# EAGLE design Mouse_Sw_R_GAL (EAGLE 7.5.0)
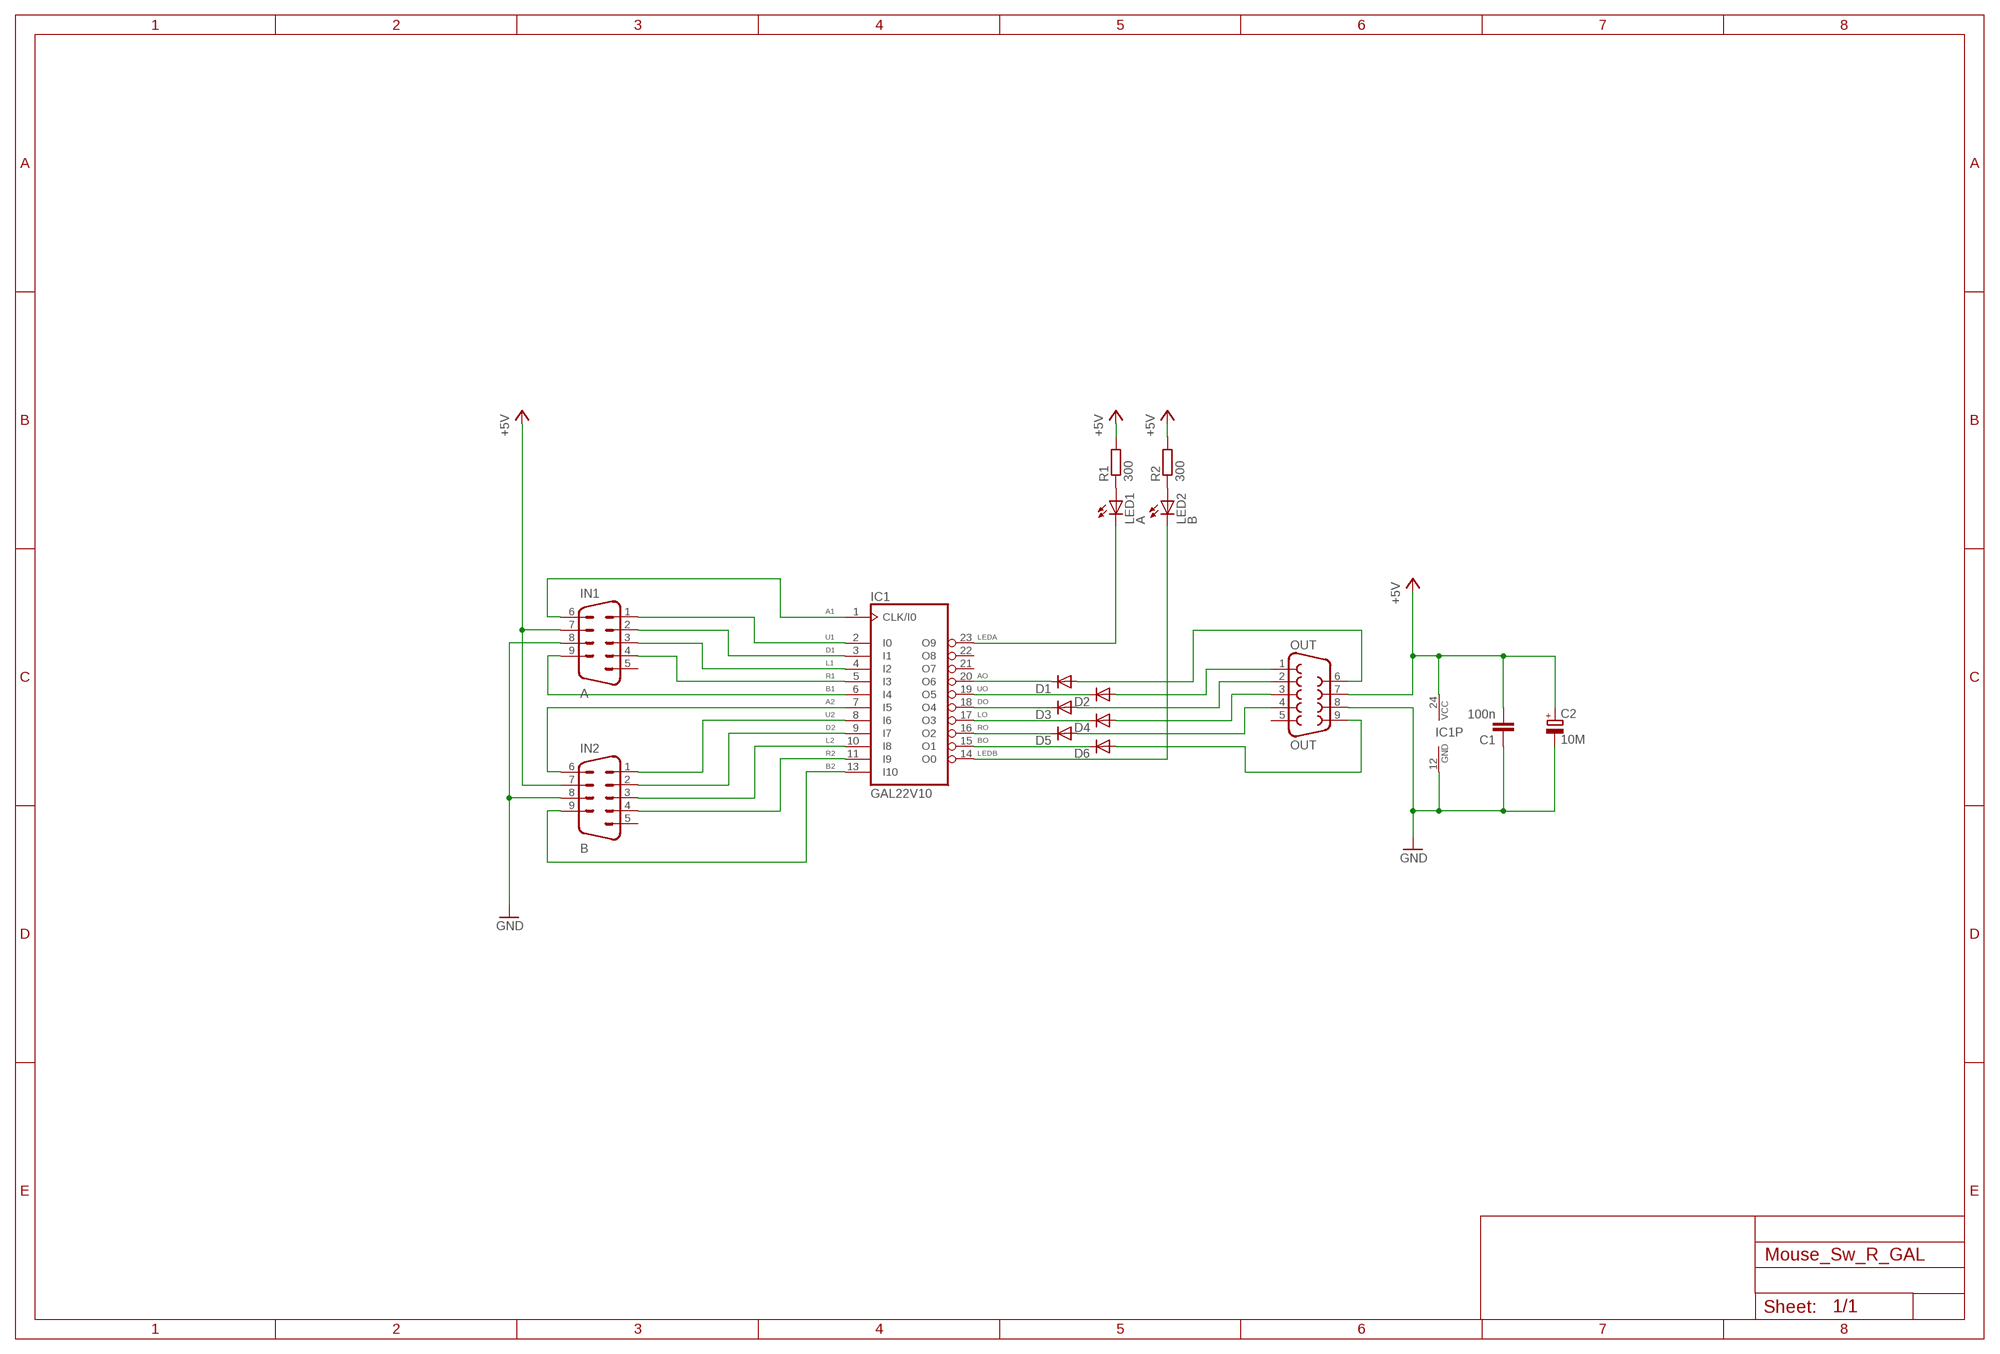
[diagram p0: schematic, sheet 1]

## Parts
C1  100n  C-EU050-024X044  [C050-024X044]
C2  10M  CPOL-EUE2.5-5  [E2,5-5]
D1  DIODE-D-5  [D-5]
D2  DIODE-D-5  [D-5]
D3  DIODE-D-5  [D-5]
D4  DIODE-D-5  [D-5]
D5  DIODE-D-5  [D-5]
D6  DIODE-D-5  [D-5]
IC1  GAL22V10  22V10  [DIL24-3]
IN1  A  M09D  [M09D]
IN2  B  M09D  [M09D]
LED1  A  LED3MM  [LED3MM]
LED2  B  LED3MM  [LED3MM]
OUT  OUT  F09D  [F09D]
R1  300  R-EU_0204/5  [0204/5]
R2  300  R-EU_0204/5  [0204/5]

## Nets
+5V: C1.2 C2.+ IC1.24(VCC) IN1.7 IN2.7 OUT.7 R1.2 R2.2
A: D1.A OUT.6
A1: IC1.1(CLK/I0) IN1.6
A2: IC1.7(I5) IN2.6
AO: D1.C IC1.20(O6)
B: D6.A OUT.9
B1: IC1.6(I4) IN1.9
B2: IC1.13(I10) IN2.9
BO: D6.C IC1.15(O1)
D: D3.A OUT.2
D1: IC1.3(I1) IN1.2
D2: IC1.9(I7) IN2.2
DO: D3.C IC1.18(O4)
GND: C1.1 C2.- IC1.12(GND) IN1.8 IN2.8 OUT.8
L: D4.A OUT.3
L1: IC1.4(I2) IN1.3
L2: IC1.10(I8) IN2.3
LEDA: IC1.23(O9) LED1.K(C)
LEDB: IC1.14(O0) LED2.K(C)
LO: D4.C IC1.17(O3)
N$22: LED1.A R1.1
N$29: LED2.A R2.1
R: D5.A OUT.4
R1: IC1.5(I3) IN1.4
R2: IC1.11(I9) IN2.4
RO: D5.C IC1.16(O2)
U: D2.A OUT.1
U1: IC1.2(I0) IN1.1
U2: IC1.8(I6) IN2.1
UO: D2.C IC1.19(O5)
Unconnected: IC1.21(O7) IC1.22(O8) IN1.5 IN2.5 OUT.5

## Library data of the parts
C1 = rcl:C-EU: CAPACITOR, European symbol
C2 = rcl:CPOL-EU: POLARIZED CAPACITOR, European symbol
D1-D6 = diode:DIODE-: DIODE
IC1 = pal:22V10: PAL; MPN: GAL22V10D-7LPN; OC_FARNELL: 1571925; OC_NEWARK: 97M0480
IN1 IN2 = con-subd:M09: SUB-D; OC_FARNELL: unknown; OC_NEWARK: unknown
LED1 LED2 = led:LED: LED
OUT = con-subd:F09: SUB-D; OC_FARNELL: unknown; OC_NEWARK: unknown
R1 R2 = rcl:R-EU_: RESISTOR, European symbol

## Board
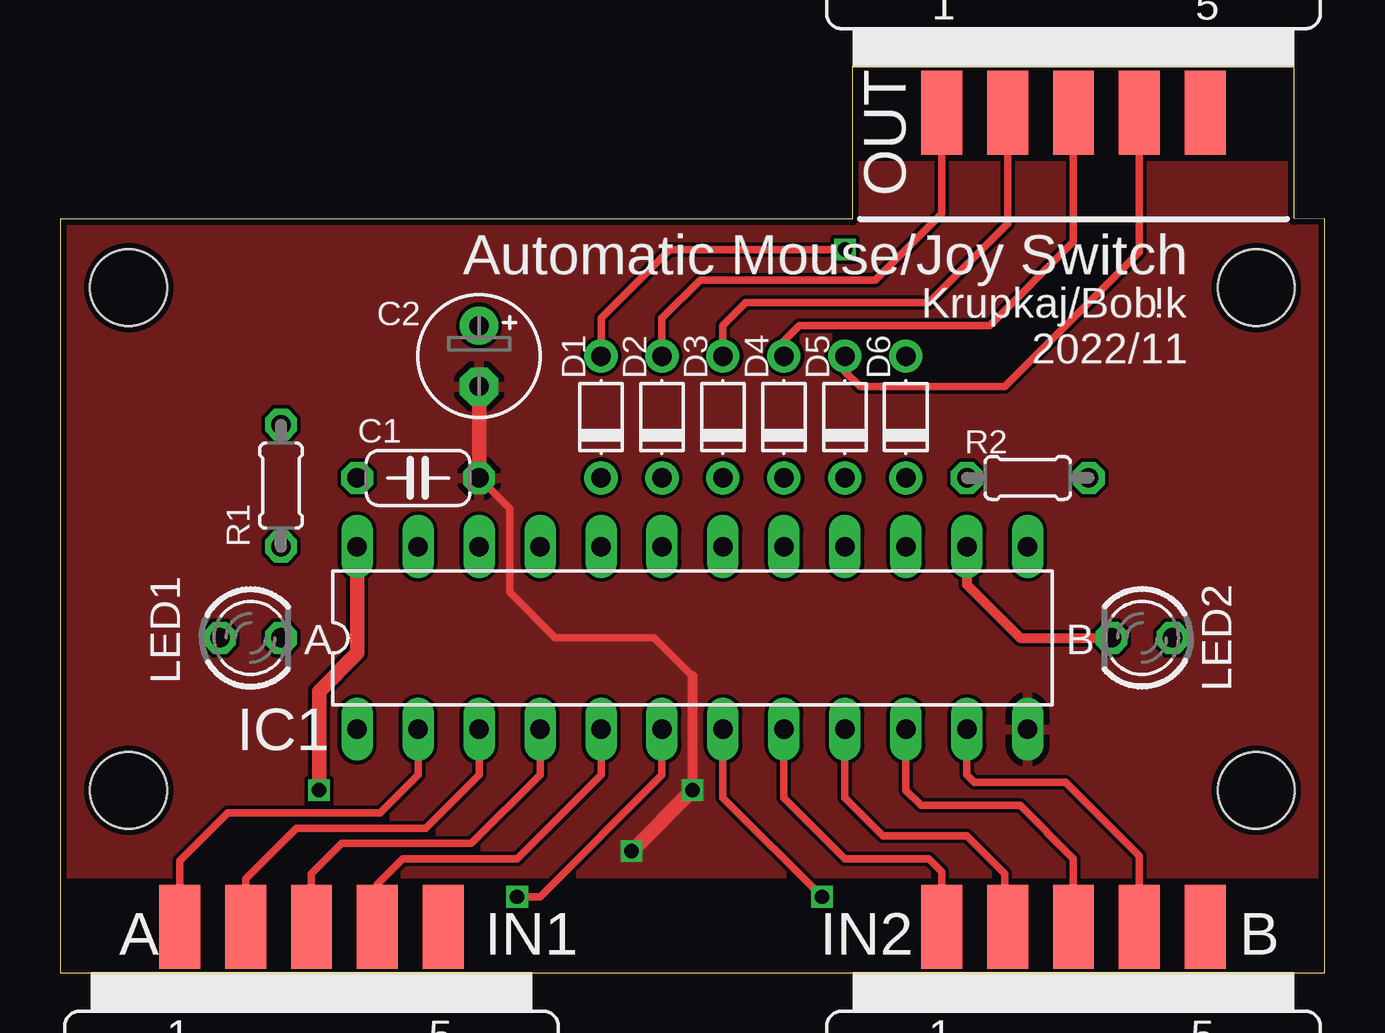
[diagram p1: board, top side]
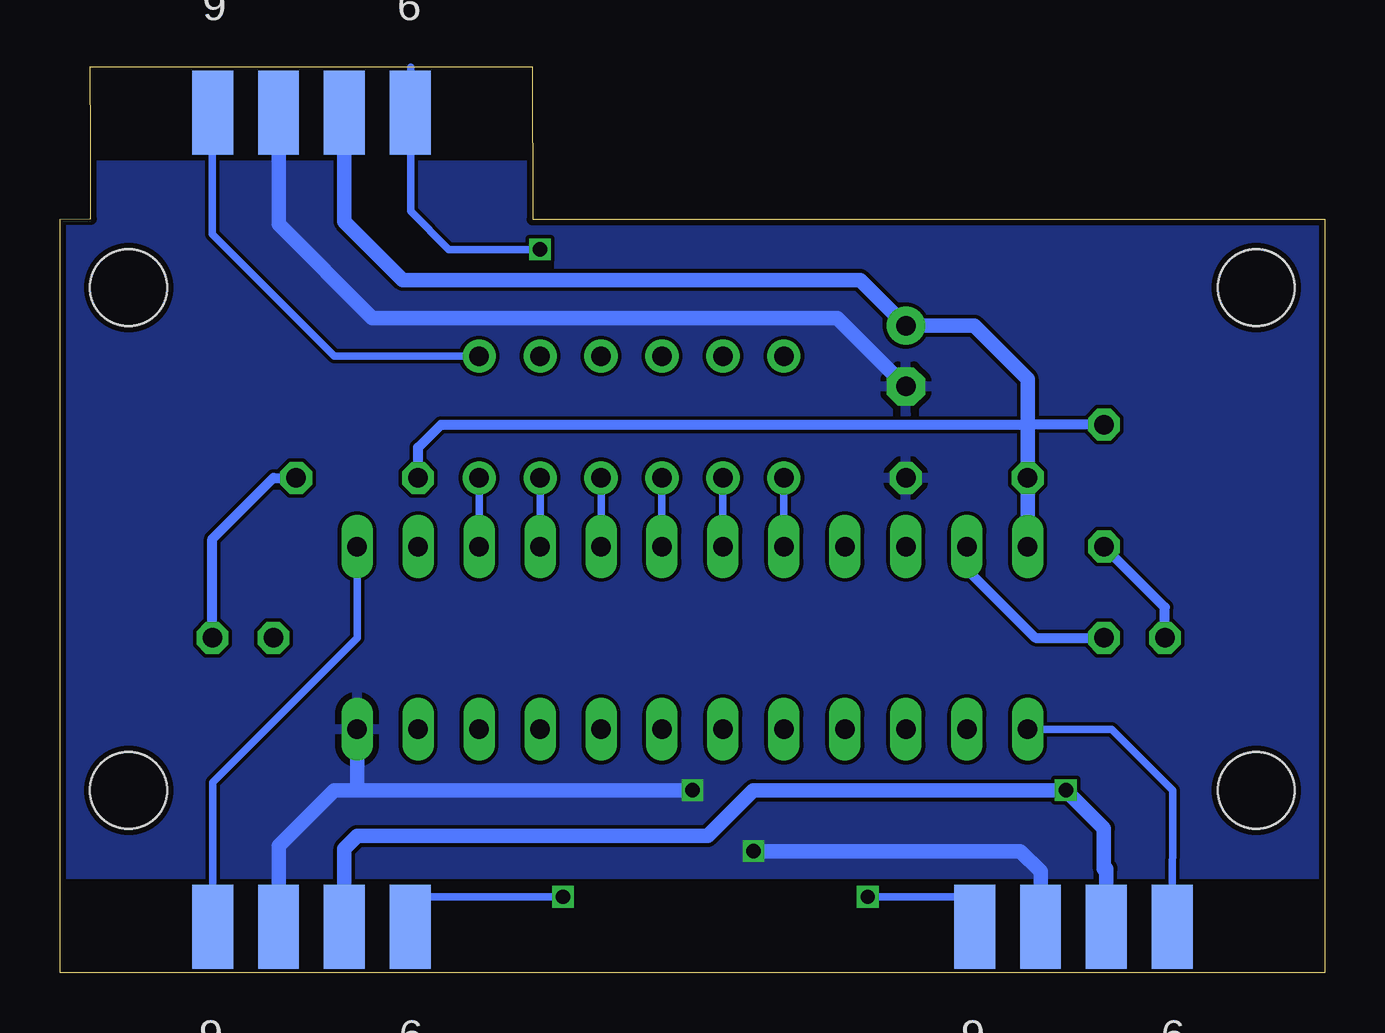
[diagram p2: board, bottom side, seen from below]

Size 52.7 x 37.78 mm. Coordinates in mm from the lower left corner, seen from the top.
Outline: 0,0 52.69,0 52.71,31.43 51.42,31.45 51.42,34.6 51.43,37.78 33.02,37.78 33.01,31.42 0,31.42 0,0
Copper layers (1*16): Top 0.035mm / dielectric 1.5mm / Bottom 0.035mm
Design rules "SeeedStudio_2layer_DRU_no_angle_20140221": minimum track width 6mil, minimum drill 12mil, track to track 6mil, track to pad 6mil, pad to pad 6mil, via to via 6mil, smd to smd 0mil, copper to edge 10mil, drill to drill 10mil, minimum pad ring 10mil, minimum via ring 6mil, stop-mask expansion 2mil, vias tented up to drill 100mil, thermal gap 10mil
Holes 3.2 mm at 49.85,7.62 2.86,7.62 2.86,28.57 49.85,28.57

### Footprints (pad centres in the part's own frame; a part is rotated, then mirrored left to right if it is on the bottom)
C050-024X044 = drill 0.813 octagon: 1 -2.54,0; 2 2.54,0
E2,5-5 = drill 0.813 pad 1.6: + -1.27,0 | drill 0.813 pad 1.6 octagon: - 1.27,0
D-5 = drill 0.813 pad 1.38: A 2.54,0; C -2.54,0
DIL24-3 = drill 0.813 long: 1 -13.97,-3.81; 2 -11.43,-3.81; 3 -8.89,-3.81; 4 -6.35,-3.81; 5 -3.81,-3.81; 6 -1.27,-3.81; 7 1.27,-3.81; 8 3.81,-3.81; 9 6.35,-3.81; 10 8.89,-3.81; 11 11.43,-3.81; 12 13.97,-3.81; 13 13.97,3.81; 14 11.43,3.81; 15 8.89,3.81; 16 6.35,3.81; 17 3.81,3.81; 18 1.27,3.81; 19 -1.27,3.81; 20 -3.81,3.81; 21 -6.35,3.81; 22 -8.89,3.81; 23 -11.43,3.81; 24 -13.97,3.81
M09D = smd 1.7 x 3.5: 1 5.486,-6.045; 2 2.743,-6.045; 3 0,-6.045; 4 -2.743,-6.045; 5 -5.486,-6.045 | smd 1.7 x 3.5 bottom: 6 4.115,-6.045; 7 1.372,-6.045; 8 -1.372,-6.045; 9 -4.115,-6.045
LED3MM = drill 0.813 octagon: A -1.27,0; K 1.27,0
F09D = smd 1.7 x 3.5: 1 -5.486,-6.045; 2 -2.743,-6.045; 3 0,-6.045; 4 2.743,-6.045; 5 5.486,-6.045 | smd 1.7 x 3.5 bottom: 6 -4.115,-6.045; 7 -1.372,-6.045; 8 1.372,-6.045; 9 4.115,-6.045
0204/5 = drill 0.813 octagon: 1 -2.54,0; 2 2.54,0

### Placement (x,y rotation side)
C1  14.92,20.64 180 top
C2  17.46,25.72 270 top
D1  22.54,23.18 90 top
D2  25.08,23.18 90 top
D3  27.62,23.18 90 top
D4  30.16,23.18 90 top
D5  32.7,23.18 90 top
D6  35.24,23.18 90 top
IC1  26.35,13.97 0 top
IN1  10.48,-4.13 180 top
IN2  42.23,-4.13 180 top
LED1  7.94,13.97 0 top
LED2  45.09,13.97 180 top
OUT  42.23,41.91 0 top
R1  9.21,20.32 90 top
R2  40.32,20.64 180 top

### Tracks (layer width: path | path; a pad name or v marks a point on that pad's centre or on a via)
+5V  (via drill 0.6)
  Top 0.61: v10.8,7.62 10.8,11.75 12.38,13.34 IC1.24
  Bottom 0.406: R2.2 37.78,21.91 36.83,22.86 12.38,22.86 R1.2
  Bottom 0.61: IN2.7 40.86,5.18 40.32,5.71 25.72,5.71 23.81,7.62 v10.8,7.62 9.21,6.03 9.21,4.34 9.11,4.34 IN1.7 | OUT.7 40.86,31.33 38.42,28.89 19.37,28.89 C2.+ 14.6,26.99 12.38,24.77 12.38,22.86 C1.2 IC1.24
A  (via drill 0.6)
  Top 0.305: D1.A 22.54,27.3 25.4,30.16 v32.7,30.16
  Bottom 0.305: OUT.6 38.1,37.76 38.1,31.75 36.51,30.16 v32.7,30.16
A1
  Bottom 0.305: IN1.6 6.36,4.14 6.35,5.4 6.35,7.62 8.89,10.16 IC1.1
A2  (via drill 0.6)
  Top 0.305: v31.75,3.17 27.62,7.3 IC1.7
  Bottom 0.305: IN2.6 38.13,3.17 v31.75,3.17
AO
  Bottom 0.305: D1.C IC1.20
B
  Bottom 0.305: OUT.9 46.35,36.17 46.35,30.8 41.28,25.72 D6.A
B1  (via drill 0.6)
  Top 0.305: v19.05,3.17 20,3.17 25.08,8.26 IC1.6
  Bottom 0.305: IN1.9 14.59,2.21 14.92,2.54 14.92,3.17 v19.05,3.17
B2
  Bottom 0.305: IN2.9 46.34,7.95 40.32,13.97 IC1.13
BO
  Bottom 0.305: IC1.15 D6.C
D
  Top 0.305: D3.A 27.62,26.99 28.57,27.94 36.2,27.94 39.48,31.23 OUT.2
D1
  Top 0.305: IN1.2 7.73,3.92 9.84,6.03 15.24,6.03 17.46,8.26 IC1.3
D2
  Top 0.305: IN2.2 39.37,2.03 39.37,4.13 37.78,5.71 34.29,5.71 32.7,7.3 IC1.9
DO
  Bottom 0.305: IC1.18 D3.C
GND  (via drill 0.6)
  Top 0.305: C1.1 18.73,19.37 18.73,15.88 20.64,13.97 24.77,13.97 26.35,12.38
  Top 0.406: 26.35,12.38 v26.35,7.62
  Top 0.61: v26.35,7.62 v23.81,5.08 | C2.- C1.1
  Bottom 0.61: v23.81,5.08 12.7,5.08 11.85,4.23 IN1.8 | OUT.8 43.6,31.22 39.69,27.3 20.32,27.3 C2.- | IN2.8 43.6,5.3 41.28,7.62 40.32,7.62 | 40.32,7.62 IC1.12 | v26.35,7.62 40.32,7.62
  pour Top: -3.17,33.66 53.98,33.66 53.98,4.13 -3.17,4.13
  pour Bottom: -2.22,33.66 55.56,33.66 56.2,4.13 -1.59,4.13
L
  Top 0.305: D4.A 30.16,26.35 30.8,26.99 38.74,26.99 42.23,30.48 OUT.3
L1
  Top 0.305: IN1.3 10.48,4.13 11.75,5.4 17.15,5.4 20,8.26 IC1.4
L2
  Top 0.305: 42.23,4.13 IN2.3 42.23,4.76 40,6.99 35.88,6.99 35.24,7.62 IC1.10
LEDA
  Bottom 0.406: IC1.23 14.92,16.83 12.06,13.97 LED1.K
LEDB
  Top 0.406: IC1.14 37.78,16.19 40,13.97 LED2.K
LO
  Bottom 0.305: IC1.17 D4.C
N$22
  Bottom 0.406: LED1.A 6.67,15.24 R1.1
N$29
  Bottom 0.406: LED2.A 46.35,18.1 43.81,20.64 R2.1
R
  Top 0.305: OUT.4 44.97,30.05 39.37,24.45 33.34,24.45 32.7,25.08 D5.A
R1
  Top 0.305: IN1.4 13.22,3.7 14.29,4.76 19.05,4.76 22.54,8.26 IC1.5
R2
  Top 0.305: IC1.11 37.78,8.26 38.1,7.94 41.91,7.94 44.97,4.88 IN2.4
RO
  Bottom 0.305: IC1.16 D5.C
U
  Top 0.305: D2.A 25.08,27.3 26.67,28.89 33.97,28.89 36.74,31.66 OUT.1
U1
  Top 0.305: IC1.2 14.92,8.26 13.33,6.67 6.98,6.67 4.99,4.67 IN1.1
U2
  Top 0.305: IN2.1 36.74,4.22 36.2,4.76 32.7,4.76 30.16,7.3 IC1.8
UO
  Bottom 0.305: D2.C IC1.19

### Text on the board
tPlace: ! | k | 2022/11
tNames: Automatic Mouse/Joy Switch | Krupkaj/Bob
